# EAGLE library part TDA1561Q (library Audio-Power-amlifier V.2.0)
The TDA1561Q is a monolithic power amplifier in a 13 lead single-in-line (SIL) plastic power package. It contains two identical 23 W amplifiers. The dissipation is minimized by switching from SE to BTL mode, only when a higher output voltage swing is needed. The device is primarily developed for car radio applications.
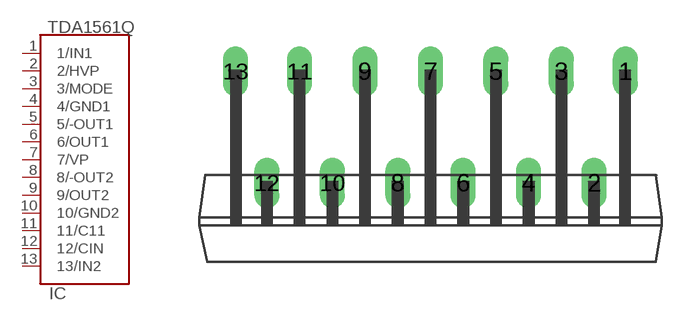
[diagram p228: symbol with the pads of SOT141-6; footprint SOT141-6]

Designator prefix IC

## TDA1561Q  [SOT141-6]
1  1/IN1  in
2  2/HVP  in
3  3/MODE  in
4  4/GND1  pwr
5  5/-OUT1  out
6  6/OUT1  out
7  7/VP  pwr
8  8/-OUT2  out
9  9/OUT2  out
10  10/GND2  pwr
11  11/C11
12  12/CIN  in
13  13/IN2  in

## Footprint SOT141-6 (pad centres in mm)
drill 0.8 long: 1 10.12,5.8; 2 8.5,0; 3 6.8,5.8; 4 5.1,0; 5 3.4,5.8; 6 1.7,0; 7 0,5.8; 8 -1.7,0; 9 -3.4,5.8; 10 -5.1,0; 11 -6.8,5.8; 12 -8.5,0; 13 -10.12,5.8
